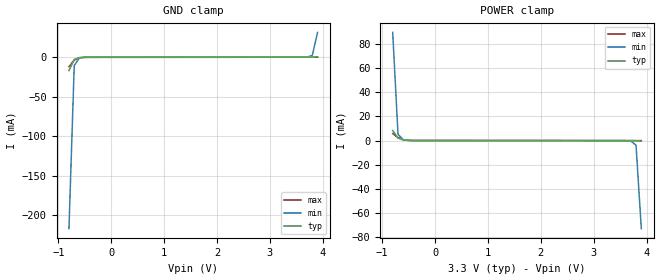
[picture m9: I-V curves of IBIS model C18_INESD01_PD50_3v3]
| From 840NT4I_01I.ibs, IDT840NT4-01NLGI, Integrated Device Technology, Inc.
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[Model] C18_INESD01_PD50_3v3
Model_type   Input
Polarity   Non-Inverting
Vinl = 0.8V
Vinh = 2.0V
|   typ   min   max
C_comp   2pF   1.5pF   2.5pF
|   typ   min   max
[Voltage range]   3.3V   3.135V   3.465V
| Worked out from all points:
|   GND clamp passes 1 mA (typ) near -0.62 V on its own axis
|   POWER clamp passes 1 mA (typ) near -0.63 V on its own axis
[GND_clamp]
|Voltage   I (typ)   I (min)   I (max)
|Note, modeling breaks down at 250mA and above.  This is well beyond the functional   |
|operating range of the device.  Should this scenario occur, catastrophic failure and   |
|possible damage to the device and/or board is of higher concern than the I-V curve   |
|behavior.  The IBIS checker will flag currents in excess of 10A with warnings.  Lines   |
|with currents in excess of 0.35 A have been commented out.  The points still remain|
|available to the user if the user desires to use them.   |
|-3.30000e+00   -3.86204e+01   -3.32347e+01   -4.76611e+01
|-3.20000e+00   -3.70319e+01   -3.19123e+01   -4.56309e+01
|-3.10000e+00   -3.54432e+01   -3.05897e+01   -4.36003e+01
|-3.00000e+00   -3.38541e+01   -2.92669e+01   -4.15694e+01
|-2.90000e+00   -3.22649e+01   -2.79439e+01   -3.95382e+01
|-2.80000e+00   -3.06753e+01   -2.66208e+01   -3.75066e+01
|-2.70000e+00   -2.90855e+01   -2.52975e+01   -3.54746e+01
|-2.60000e+00   -2.74954e+01   -2.39740e+01   -3.34423e+01
|-2.50000e+00   -2.59051e+01   -2.26503e+01   -3.14096e+01
|-2.40000e+00   -2.43145e+01   -2.13264e+01   -2.93765e+01
|-2.30000e+00   -2.27236e+01   -2.00024e+01   -2.73430e+01
|-2.20000e+00   -2.11325e+01   -1.86782e+01   -2.53091e+01
|-2.10000e+00   -1.95411e+01   -1.73539e+01   -2.32749e+01
|-2.00000e+00   -1.79495e+01   -1.60295e+01   -2.12403e+01
|-1.90000e+00   -1.63577e+01   -1.47050e+01   -1.92054e+01
|-1.80000e+00   -1.47658e+01   -1.33803e+01   -1.71701e+01
|-1.70000e+00   -1.31736e+01   -1.20557e+01   -1.51345e+01
|-1.60000e+00   -1.15814e+01   -1.07310e+01   -1.30986e+01
|-1.50000e+00   -9.98912e+00   -9.40639e+00   -1.10625e+01
|-1.40000e+00   -8.39688e+00   -8.08189e+00   -9.02622e+00
|-1.30000e+00   -6.80479e+00   -6.75760e+00   -6.98988e+00
|-1.20000e+00   -5.21297e+00   -5.43362e+00   -4.95364e+00
|-1.10000e+00   -3.62164e+00   -4.11011e+00   -2.91772e+00
|-1.00000e+00   -2.03108e+00   -2.78728e+00   -8.82465e-01
|-9.00000e-01   -4.41714e-01   -1.46545e+00   -3.28065e-02
-800mV    -16.87mA   -217.3mA   -11.98mA
-700mV    -2.708mA   -10.29mA   -3.634mA
-600mV    -453.3uA   -698.6uA   -527.7uA
3.7V      77.31uA    339.6uA    78.55uA
3.8V      131.3uA    2.343mA    80.79uA
3.9V      567.9uA    31.56mA    88.81uA
| 4.00000e+00   2.05554e-03   6.20114e-01   2.19760e-04
| 4.10000e+00   8.34754e-03   2.01524e+00   1.17235e-03
| 4.20000e+00   1.76646e-01   3.41078e+00   3.53831e-03
| 4.30000e+00   1.69641e+00   4.80670e+00   7.24157e-03
| 4.40000e+00   3.37317e+00   6.20296e+00   3.18215e-02
| 4.50000e+00   5.05036e+00   7.59952e+00   1.22067e+00
| 4.60000e+00   6.72794e+00   8.99637e+00   3.36524e+00
| 4.70000e+00   8.40586e+00   1.03935e+01   5.51029e+00
| 4.80000e+00   1.00841e+01   1.17909e+01   7.65577e+00
| 4.90000e+00   1.17626e+01   1.31886e+01   9.80161e+00
| 5.00000e+00   1.34414e+01   1.45865e+01   1.19478e+01
| 5.10000e+00   1.51205e+01   1.59848e+01   1.40942e+01
| 5.20000e+00   1.67998e+01   1.73833e+01   1.62410e+01
| 5.30000e+00   1.84795e+01   1.87822e+01   1.83880e+01
| 5.40000e+00   2.01595e+01   2.01815e+01   2.05353e+01
| 5.50000e+00   2.18398e+01   2.15812e+01   2.26828e+01
| 5.60000e+00   2.35204e+01   2.29814e+01   2.48307e+01
| 5.70000e+00   2.52015e+01   2.43821e+01   2.69789e+01
| 5.80000e+00   2.68830e+01   2.57834e+01   2.91275e+01
| 5.90000e+00   2.85651e+01   2.71855e+01   3.12764e+01
| 6.00000e+00   3.02478e+01   2.85884e+01   3.34258e+01
| 6.10000e+00   3.19311e+01   2.99923e+01   3.55757e+01
| 6.20000e+00   3.36153e+01   3.13975e+01   3.77262e+01
| 6.30000e+00   3.53004e+01   3.28040e+01   3.98773e+01
| 6.40000e+00   3.69866e+01   3.42122e+01   4.20293e+01
| 6.50000e+00   3.86741e+01   3.56225e+01   4.41821e+01
| 6.60000e+00   4.03632e+01   3.70351e+01   4.63360e+01
[Power_clamp]
|Voltage   I (typ)   I (min)   I (max)
|Note, modeling breaks down at 250mA and above.  This is well beyond the functional   |
|operating range of the device.  Should this scenario occur, catastrophic failure and   |
|possible damage to the device and/or board is of higher concern than the I-V curve   |
|behavior.  The IBIS checker will flag currents in excess of 10A with warnings.  Lines   |
|with currents in excess of 0.35 A have been commented out.  The points still remain|
|available to the user if the user desires to use them.   |
|-3.30000e+00   4.03632e+01   3.47056e+01   4.98927e+01
|-3.20000e+00   3.86741e+01   3.32967e+01   4.77366e+01
|-3.10000e+00   3.69866e+01   3.18896e+01   4.55820e+01
|-3.00000e+00   3.53004e+01   3.04840e+01   4.34285e+01
|-2.90000e+00   3.36153e+01   2.90797e+01   4.12760e+01
|-2.80000e+00   3.19311e+01   2.76764e+01   3.91243e+01
|-2.70000e+00   3.02478e+01   2.62741e+01   3.69734e+01
|-2.60000e+00   2.85651e+01   2.48725e+01   3.48232e+01
|-2.50000e+00   2.68830e+01   2.34715e+01   3.26735e+01
|-2.40000e+00   2.52015e+01   2.20712e+01   3.05242e+01
|-2.30000e+00   2.35204e+01   2.06713e+01   2.83754e+01
|-2.20000e+00   2.18398e+01   1.92719e+01   2.62270e+01
|-2.10000e+00   2.01595e+01   1.78729e+01   2.40789e+01
|-2.00000e+00   1.84795e+01   1.64742e+01   2.19312e+01
|-1.90000e+00   1.67998e+01   1.50759e+01   1.97837e+01
|-1.80000e+00   1.51205e+01   1.36778e+01   1.76365e+01
|-1.70000e+00   1.34414e+01   1.22800e+01   1.54896e+01
|-1.60000e+00   1.17626e+01   1.08826e+01   1.33429e+01
|-1.50000e+00   1.00841e+01   9.48534e+00   1.11966e+01
|-1.40000e+00   8.40586e+00   8.08839e+00   9.05053e+00
|-1.30000e+00   6.72794e+00   6.69172e+00   6.90481e+00
|-1.20000e+00   5.05036e+00   5.29536e+00   4.75947e+00
|-1.10000e+00   3.37317e+00   3.89932e+00   2.61458e+00
|-1.00000e+00   1.69641e+00   2.50363e+00   4.70211e-01
|-9.00000e-01   1.76646e-01   1.10835e+00   1.36706e-02
-800mV    8.348mA    89.38mA    5.753mA
-700mV    2.056mA    5.347mA    2.559mA
-600mV    567.9uA    633.8uA    683uA
-400mV    77.31uA    71.56uA    83.7uA
3.7V      -11.1uA    -299.6uA   -4.991uA
3.8V      -55.7uA    -3.825mA   -7.215uA
3.9V      -453.3uA   -72.73mA   -13.73uA
